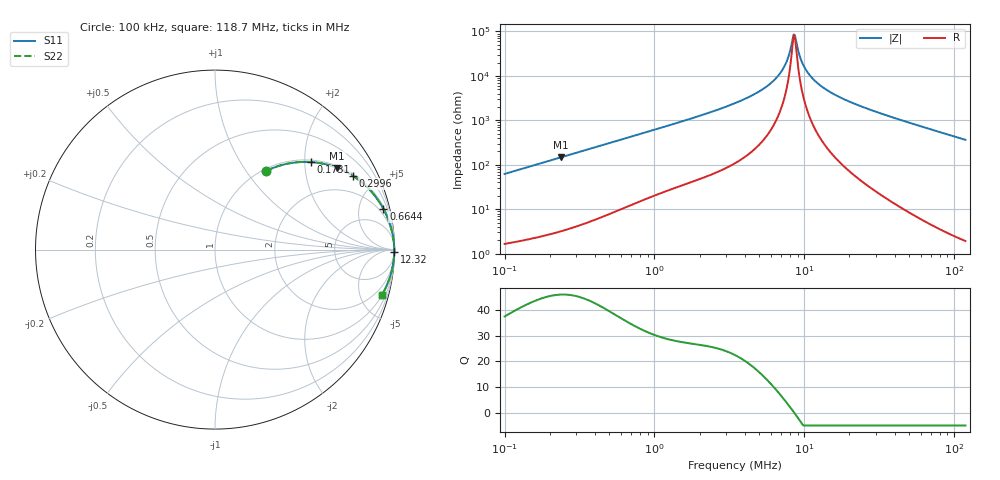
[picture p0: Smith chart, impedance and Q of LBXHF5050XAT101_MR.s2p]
! LBXHF5050XAT101_MR  S-PARAMETER MODEL  ( General Type )
! Model Generated by TAIYO YUDEN Corporation (http://www.ty-top.com)
! Version 1.0
! TAIYO YUDEN Control No. 201105NI43SB-FBB
! Copyright(c) 2020 TAIYO YUDEN CO.,LTD. All Rights Reserved.
! Product Description (link to TY-COMPAS)
! https://ds.yuden.co.jp/TYCOMPAS/or/detail?pn=LBXHF5050XAT101MMR&u=M
! Products Name : Inductors
! Characteristics :
!  Inductance : 100 uH , SRF(min) : 6.0 MHz , DC Resistance(max) : 0.733 Ohm
!  Rated Current : Saturation :550 mA , Temp Rise : 450 mA
!  Case Size : 5.0 x 5.0 / 0.197 x 0.197 [mm/inch] , Thickness : 3.1 / 0.122 [mm/inch]
!  (Conditions: Temperature = 25 degC , DC Bias Current/Voltage = 0A / 0V)
! External Node Assignments :
!  1  o---GGG---o  2
! GND o---------o GND
! Frequency Range : 0.1MHz  -  118.695536MHz  [ 402 STEP ]
# MHz S RI R 50
! Freq[MHz].  S11 Real  S11 Imag  S21 Real  S21 Imag  S12 Real  S12 Imag  S22 Real  S22 Imag
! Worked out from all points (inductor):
!   401 points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, 100 kHz to 118.7 MHz, reference 50 ohm
!   read as one part in series: L = 98.9 uH near 103.6 kHz
!   highest Q = 46.1 at 238 kHz (marker M1), where L = 98.6 uH
!   self-resonance near 8.496 MHz
!   S11 on the Smith chart (normalised r, x): 100 kHz: 1.03, +1.25; 173.1 kHz: 1.05, +2.15; 299.6 kHz: 1.08, +3.71; 664.4 kHz: 1.23, +8.18; 12.32 MHz: open; 118.7 MHz: 1.04, -7.30
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0.1  0.2849 0.4383  0.7151 -0.4383  0.7151 -0.4383  0.2849 0.4383
0.173089  0.5349 0.4877  0.4651 -0.4877  0.4651 -0.4877  0.5349 0.4877
0.238023  0.6812 0.4553  0.3188 -0.4553  0.3188 -0.4553  0.6812 0.4553
0.299597  0.7696 0.4103  0.2304 -0.4103  0.2304 -0.4103  0.7696 0.4103
0.327316  0.7985 0.3901  0.2015 -0.3901  0.2015 -0.3901  0.7985 0.3901
0.664372  0.938 0.2274  0.062 -0.2274  0.062 -0.2274  0.938 0.2274
1.07136  0.9729 0.1465  0.0271 -0.1465  0.0271 -0.1465  0.9729 0.1465
3.445222  0.9965 0.0408  0.00349 -0.0408  0.00349 -0.0408  0.9965 0.0408
5.085236  0.9981 0.0214  0.00185 -0.0214  0.00185 -0.0214  0.9981 0.0214
6.515028  0.9986 0.0109  0.00136 -0.0109  0.00136 -0.0109  0.9986 0.0109
7.505938  0.9988 0.00516  0.00121 -0.00516  0.00121 -0.00516  0.9988 0.00516
7.915224  0.9988 0.00305  0.00117 -0.00305  0.00117 -0.00305  0.9988 0.00305
8.346829  0.9989 0.000953  0.00114 -0.000953  0.00114 -0.000953  0.9989 0.000953
8.495864  0.9989 0.000253  0.00114 -0.000253  0.00114 -0.000253  0.9989 0.000253
8.801967  0.9989 -0.00115  0.00113 0.00115  0.00113 0.00115  0.9989 -0.00115
9.281924  0.9989 -0.00325  0.00112 0.00325  0.00112 0.00325  0.9989 -0.00325
9.788052  0.9989 -0.00536  0.00113 0.00536  0.00113 0.00536  0.9989 -0.00536
11.27678  0.9988 -0.0111  0.0012 0.0111  0.0012 0.0111  0.9988 -0.0111
12.32013  0.9987 -0.0148  0.00128 0.0148  0.00128 0.0148  0.9987 -0.0148
18.50953  0.9978 -0.0337  0.00216 0.0337  0.00216 0.0337  0.9978 -0.0337
36.91074  0.9925 -0.0803  0.00754 0.0803  0.00754 0.0803  0.9925 -0.0803
118.6955  0.929 -0.2541  0.071 0.2541  0.071 0.2541  0.929 -0.2541
